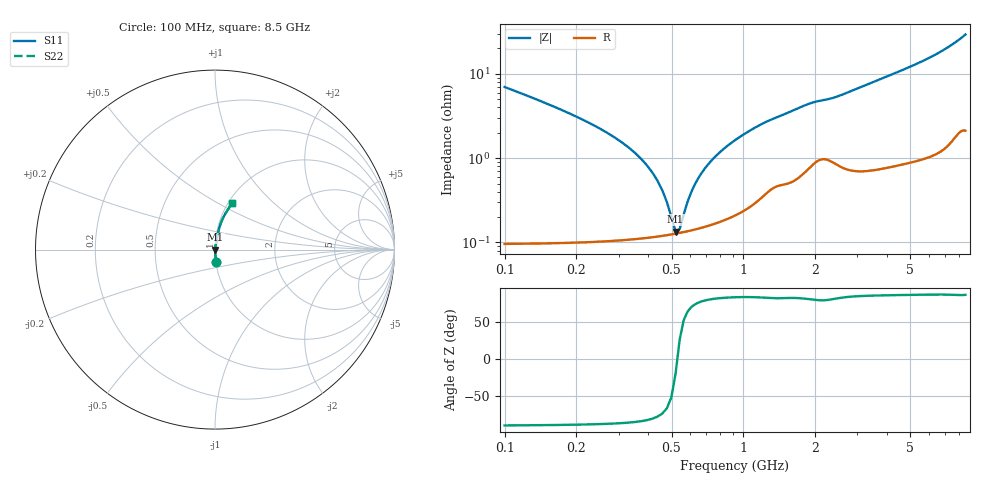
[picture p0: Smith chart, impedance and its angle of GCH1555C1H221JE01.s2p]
!Murata Part Number: GCH1555C1H221JE01
!These Parameters are Measured in Series Mode Connection
!Data Generated on Jun 19, 2026
!  o--ll--o
!Port1  Port2
!  o------o
!Operation Temp=25[degC], DC Bias Voltage=0[V]
!Freq. Start=100[MHz] Stop=9[GHz] 401[Steps]
# Hz S RI R 50
!Freq.(Hz) S11(Real) S11(Imag) S21(Real) S21(Imag) S12(Real) S12(Imag) S22(Real) S22(Imag)
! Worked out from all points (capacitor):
!   401 points, 100 MHz to 8.5 GHz, reference 50 ohm
!   read as one part in series: C = 220 pF near 142 MHz
!   lowest |Z| = 135 mohm at 520 MHz (marker M1)
!   series resonance near 528.7 MHz, so ESL is about 410 pH
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1e8  0.00579 -0.0693  0.9942 0.0693  0.9942 0.0693  0.00579 -0.0693
1.42e8  0.0032 -0.0471  0.9968 0.0471  0.9968 0.0471  0.0032 -0.0471
3.73e8  0.00121 -0.00973  0.9988 0.00973  0.9988 0.00973  0.00121 -0.00973
4.36e8  0.0012 -0.0053  0.9988 0.0053  0.9988 0.0053  0.0012 -0.0053
4.99e8  0.00125 -0.00158  0.9988 0.00158  0.9988 0.00158  0.00125 -0.00158
5.2e8  0.00127 -0.000449  0.9987 0.000449  0.9987 0.000449  0.00127 -0.000449
5.41e8  0.0013 0.000634  0.9987 -0.000634  0.9987 -0.000634  0.0013 0.000634
5.62e8  0.00133 0.00168  0.9987 -0.00168  0.9987 -0.00168  0.00133 0.00168
6.25e8  0.00144 0.00461  0.9986 -0.00461  0.9986 -0.00461  0.00144 0.00461
6.67e8  0.00153 0.00643  0.9985 -0.00643  0.9985 -0.00643  0.00153 0.00643
7.3e8  0.00169 0.00901  0.9983 -0.00901  0.9983 -0.00901  0.00169 0.00901
8.35e8  0.00201 0.013  0.998 -0.013  0.998 -0.013  0.00201 0.013
9.61e8  0.00251 0.0175  0.9975 -0.0175  0.9975 -0.0175  0.00251 0.0175
1.129e9  0.00351 0.023  0.9965 -0.023  0.9965 -0.023  0.00351 0.023
1.276e9  0.00476 0.0273  0.9952 -0.0273  0.9952 -0.0273  0.00476 0.0273
1.507e9  0.006 0.033  0.994 -0.033  0.994 -0.033  0.006 0.033
1.927e9  0.00995 0.0436  0.9901 -0.0436  0.9901 -0.0436  0.00995 0.0436
2.914e9  0.011 0.0632  0.989 -0.0632  0.989 -0.0632  0.011 0.0632
4.3e9  0.0178 0.0986  0.9822 -0.0986  0.9822 -0.0986  0.0178 0.0986
5.707e9  0.0294 0.1384  0.9706 -0.1384  0.9706 -0.1384  0.0294 0.1384
7.114e9  0.0512 0.1892  0.9488 -0.1892  0.9488 -0.1892  0.0512 0.1892
8.5e9  0.0946 0.2587  0.9054 -0.2587  0.9054 -0.2587  0.0946 0.2587
